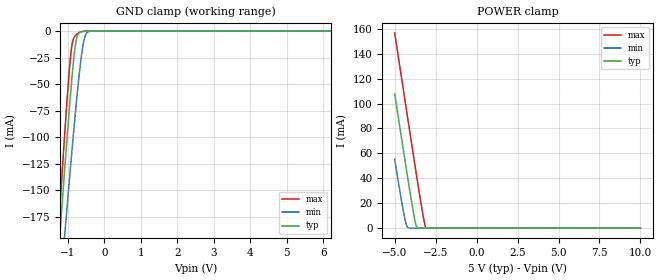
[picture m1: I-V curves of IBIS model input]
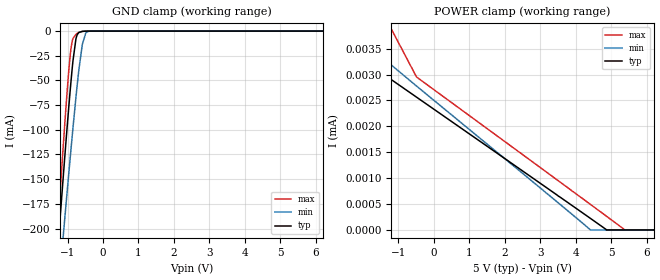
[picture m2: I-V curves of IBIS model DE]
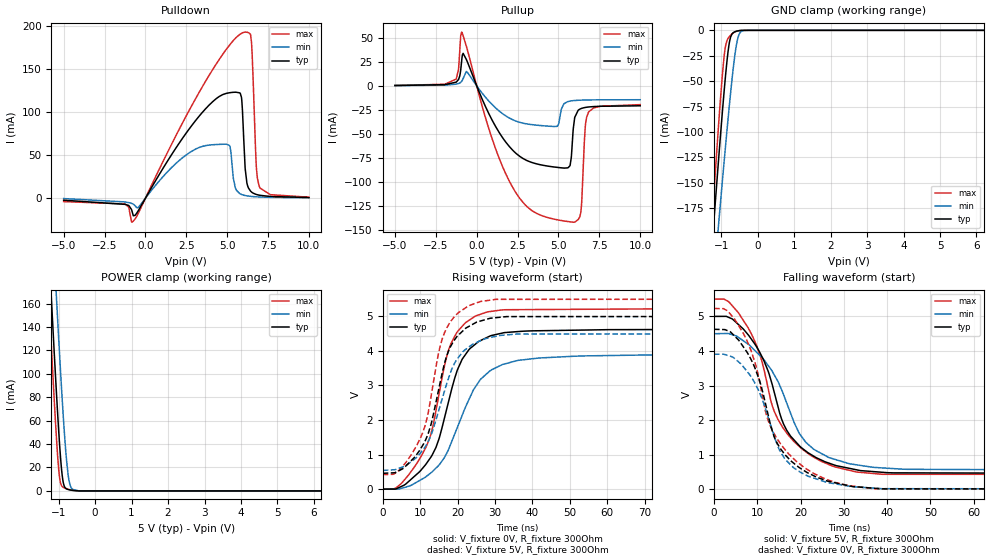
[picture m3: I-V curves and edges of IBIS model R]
|Texas Instruments Incorporated
| THVD1500 5-V RS-485 Transceivers With +/-16-kV IEC ESD Protection
| Marketing part#   Digital Voltage Range   Package-type   #pins
| THVD1500D   4.5V-5.5V   SOIC   8
| THVD1500DGK   4.5V-5.5V   VSSOP   8
[IBIS Ver]   4.1
[File name]   thvd1500.ibs
[Date]   06/22/2017
[File Rev]   1.0
[Source]
| Texas Instruments Incorporated.
| Analog-eLab Design Center, HPA
| 12500 TI Blvd
| Dallas, TX -75243
[Notes]
| Rev 1.0: 06/22/2017
| - Initial version of the model
| - Model generated from simulations in SPECTRE
| - Model matched to SPICE simulation
| - C_comp although listed in numerical order of value are
|   obtained from varying PVT conditions. For PVT conditions for
|   each specific value refer the buffer description under
|   respective [Model]. IBIS model user is responsible for using
|   appropriate C_comp to simulate for Signal Integrity.
| - Warnings regarding combined Non-monotonicity of various models
|   have been reviewed and considered minor and can be ignored.
| - Connect 1uF capacitor at the common mode node or bias the common mode
|   node to common mode voltage (Vcm= Vdd/2) for "diff" model.
[Disclaimer]
| This model is designed as an aid for customers of Texas Instruments.
| TI and its licensors and suppliers make no warranties, either expressed
| or implied, with respect to this  model, including the warranties of
| merchantability or fitness for a particular purpose. The model is
| provided solely on an "as is" basis. The entire risk as to its quality
| and performance is with the customer.
[Copyright]
(C) Copyright 2017 Texas Instruments Incorporated.All rights reserved.
|   THVD1500D
[Component]   THVD1500D
[Manufacturer]  TI
[Package]   |8 SOIC - D package
|   typ   min   max
R_pkg   0.10253625   0.06439   0.14266
L_pkg   2.75548625nH   2.22171nH   3.36255nH
C_pkg   0.4486575pF   0.38224pF   0.53208pF
[Pin]  signal_name model_name   R_pin   L_pin   C_pin
1   R   R   0.14266   3.36255nH   0.45815pF
2   _RE   input   0.12915   2.66262nH   0.38676pF
3   DE   DE   0.12314   2.56565nH   0.38224pF
4   D   input   0.13372   3.21721nH   0.45009pF
5   GND   gnd   0.0779   2.80108nH   0.51775pF
6   A   diff   0.06439   2.22171nH   0.42942pF
7   B   diff   0.06577   2.26041nH   0.43277pF
8   VCC   power   0.08356   2.95266nH   0.53208pF
[Diff Pin]  inv_pin  vdiff  tdelay_typ tdelay_min tdelay_max
6   7   0.2   NA   NA   NA
|   THVD1500DGK
[Component]   THVD1500DGK
[Manufacturer]  TI
[Package]   |8 VSSOP - DGK package
|   typ   min   max
R_pkg   0   0   0
L_pkg   0   0   0
C_pkg   0   0   0
[Pin]  signal_name model_name   R_pin   L_pin   C_pin
1   R   R   NA   NA   NA
2   _RE   input   NA   NA   NA
3   DE   DE   NA   NA   NA
4   D   input   NA   NA   NA
5   GND   gnd   NA   NA   NA
6   A   diff   NA   NA   NA
7   B   diff   NA   NA   NA
8   VCC   power   NA   NA   NA
[Diff Pin]  inv_pin  vdiff  tdelay_typ tdelay_min tdelay_max
6   7   0.2   NA   NA   NA
| Models and submodels in the file (4): input (Input), DE (Input), R (3-state), diff (I/O)
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|   input Model
[Model]   input
Model_type   Input
Vinl = 0.5
Vinh = 4.5
|   typ   min   max
C_comp   2.23689E-12   2.18605E-12   2.33152E-12
[Model spec]
|subparameter
Vinl   0.5   0.45   0.55
Vinh   4.5   4.05   4.95
| Where Nom  PVT is Nominal Process, 5V, 27C
|   Fast PVT is Strong Process,  5.5V, -40C
|   Slow PVT is Weak Process,   4.5, 150C
[Voltage Range]   5   4.5   5.5
|Junction Temperature
[Temperature Range]   27   150   -40
[Power Clamp Reference]   5   4.5   5.5
[GND Clamp Reference]   0   0   0
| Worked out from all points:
|   GND clamp passes 1 mA (typ) near -0.65 V on its own axis
|   POWER clamp passes 1 mA (typ) near -3.66 V on its own axis
[GND Clamp]
|   Voltage   I(typ)   I(min)   I(max)
-5V       -2.085A    -1.893A    -2.324A
-1.25V    -208.4mA   -261mA     -185mA
-1.13V    -151.6mA   -211.2mA   -120.8mA
-1.07V    -123.8mA   -186.6mA   -89.87mA
-965mV    -76.9mA    -144.2mA   -40.07mA
-905mV    -51.84mA   -120.5mA   -18.16mA
-845mV    -29.36mA   -97.32mA   -7.284mA
-770mV    -9.1mA     -69.52mA   -3.504mA
-635mV    -678.5uA   -25.82mA   -708.8uA
-530mV    -118.1uA   -5.338mA   -104.9uA
-410mV    -14.01uA   -325uA     -9.602uA
10V       0A         0A         0A
[POWER Clamp]
|   Voltage   I(typ)   I(min)   I(max)
-5V       107.7mA    55.36mA    156.7mA
-4.55V    69.33mA    19.37mA    117.8mA
-4.415V   57.93mA    9.756mA    106.2mA
-4.295V   47.87mA    3.03mA     95.86mA
-4.16V    36.66mA    210uA      84.27mA
-3.875V   13.93mA    182.7nA    59.93mA
-3.725V   3.778mA    29.3nA     47.22mA
-3.605V   201.6uA    20.98nA    37.14mA
-3.275V   0A         7.077nA    10.49mA
-3.17V    0A         3.417nA    3.331mA
-3.08V    0A         522.7pA    241.1uA
10V       0A         0A         0A
|   DE Model
[Model]   DE
Model_type   Input
Vinl = 0.5
Vinh = 4.5
|   typ   min   max
C_comp   2.23689E-12   2.18605E-12   2.33152E-12
[Model spec]
|subparameter
Vinl   0.5   0.45   0.55
Vinh   4.5   4.05   4.95
| Where Nom  PVT is Nominal Process, 5V, 27C
|   Fast PVT is Strong Process,  5.5V, -40C
|   Slow PVT is Weak Process,   4.5, 150C
[Voltage Range]   5   4.5   5.5
|Junction Temperature
[Temperature Range]   27   150   -40
[Power Clamp Reference]   5   4.5   5.5
[GND Clamp Reference]   0   0   0
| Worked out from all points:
|   GND clamp passes 1 mA (typ) near -0.64 V on its own axis
[GND Clamp]
|   Voltage   I(typ)   I(min)   I(max)
-3.5V     -1.328A    -1.234A    -1.462A
-1.28V    -222.7mA   -273.5mA   -201.3mA
-1.088V   -132.1mA   -193.9mA   -99.04mA
-992mV    -88.68mA   -155mA     -52.01mA
-920mV    -57.92mA   -126.3mA   -22.8mA
-860mV    -34.63mA   -103mA     -8.912mA
-764mV    -8.061mA   -67.37mA   -3.317mA
-680mV    -1.448mA   -39.02mA   -1.343mA
-584mV    -294.7uA   -13.67mA   -295.3uA
-488mV    -54.4uA    -2.137mA   -42.87uA
-380mV    -6.239uA   -154.1uA   -3.22uA
8.5V      0A         0A         0A
[POWER Clamp]
|   Voltage   I(typ)   I(min)   I(max)
-3.5V     7.22uA     4.553uA    28.19mA
-3.164V   3.836uA    4.309uA    2.93mA
-2.984V   3.751uA    4.202uA    6.205uA
-488mV    2.563uA    2.778uA    2.952uA
4.408V    226.7nA    4.981nA    497.3nA
4.876V    139pA      0A         261nA
5.404V    0A         0A         0A
8.5V      0A         0A         0A
|   R Model
[Model]   R
Model_type   3-state
Polarity   Non-Inverting
Vmeas = 2.5
Vref = 0
Cref = 2pF
Rref = 100000
|   typ   min   max
C_comp   3.78133E-12   3.67829E-12   3.86963E-12
| Where Nom  PVT is Nominal Process, 5V, 27C
|   Fast PVT is Strong Process,  5.5V, -40C
|   Slow PVT is Weak Process,   4.5, 150C
[Voltage Range]   5   4.5   5.5
|Junction Temperature
[Temperature Range]   27   150   -40
[Pullup Reference]   5   4.5   5.5
[Pulldown Reference]   0   0   -0
[Power Clamp Reference]   5   4.5   5.5
[GND Clamp Reference]   0   0   0
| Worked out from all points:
|   slope of the pulldown table from 0 to 0.75 V, typ, clamps not added: 30.6 ohm
|   slope of the pullup table from 0 to 0.75 V, typ, clamps not added: 25.6 ohm
|   GND clamp passes 1 mA (typ) near -0.60 V on its own axis
|   POWER clamp passes 1 mA (typ) near -0.71 V on its own axis
|   falling waveform, V_fixture 5V, R_fixture 300Ohm: 20-80 % time 8.94ns typ, 9.65ns min, 9.39ns max; typ from 5 V to 0.459 V
|   rising waveform, V_fixture 0V, R_fixture 300Ohm: 20-80 % time 8.13ns typ, 10.2ns min, 7.4ns max; typ from 0 V to 4.63 V
|   rising waveform, V_fixture 5V, R_fixture 300Ohm: 20-80 % time 6.78ns typ, 7.64ns min, 6.49ns max; typ from 0.459 V to 5 V
|   falling waveform, V_fixture 0V, R_fixture 300Ohm: 20-80 % time 8.18ns typ, 7.91ns min, 9.06ns max; typ from 4.63 V to 0 V
[Pulldown]
|   Voltage   I(typ)   I(min)   I(max)
-5V       -2.285mA   -396.6uA   -3.911mA
-740mV    -20.39mA   -6.868mA   -26.54mA
4.735V    120.5mA    62.74mA    167.5mA
5.17V     122.7mA    60.06mA    178.6mA
5.5V      123.2mA    12.2mA     185.8mA
5.8V      122mA      5.077mA    190.7mA
5.905V    111.2mA    4.177mA    191.9mA
6.1V      34.79mA    3.13mA     193.1mA
6.49V     7.213mA    2.073mA    180.9mA
6.775V    4.462mA    1.659mA    39.69mA
6.955V    3.589mA    1.472mA    14.28mA
10V       821.4uA    503.4uA    1.196mA
[GND Clamp]
|   Voltage   I(typ)   I(min)   I(max)
-5V       -2.098A    -1.919A    -2.329A
-1.445V   -305.1mA   -348.1mA   -293.5mA
-1.25V    -210.4mA   -265mA     -186.2mA
-1.235V   -203.2mA   -258.6mA   -178mA
-1.07V    -125.5mA   -189.5mA   -91.17mA
-965mV    -78.34mA   -146.6mA   -41.78mA
-905mV    -53.2mA    -122.6mA   -20.57mA
-770mV    -10.57mA   -70.95mA   -5.896mA
-605mV    -1.093mA   -18.95mA   -1.249mA
-500mV    -276.7uA   -3.145mA   -267.2uA
-365mV    -21.88uA   -163.3uA   -12.63uA
10V       0A         0A         0A
[Pullup]
|   Voltage   I(typ)   I(min)   I(max)
-5V       291.5uA    198.8uA    370.4uA
-1.25V    3.835mA    1.712mA    7.075mA
-920mV    25.99mA    4.642mA    55.98mA
2.215V    -67.34mA   -35.47mA   -106.3mA
4.915V    -84.98mA   -42.24mA   -139.6mA
5.575V    -85.45mA   -16.44mA   -141.4mA
5.785V    -74.76mA   -15.7mA    -141.9mA
5.905V    -44.88mA   -15.45mA   -142.1mA
6.37V     -23.82mA   -14.95mA   -132mA
6.64V     -22.56mA   -14.81mA   -42.7mA
6.835V    -22.09mA   -14.74mA   -27.57mA
10V       -20.84mA   -14.52mA   -19.61mA
[POWER Clamp]
|   Voltage   I(typ)   I(min)   I(max)
-5V       2.649A     2.722A     2.615A
-1.415V   296.9mA    380.3mA    256.3mA
-1.25V    194.4mA    278mA      153.3mA
-1.175V   149mA      232.4mA    108.2mA
-1.07V    88.28mA    170mA      49.46mA
-995mV    48.91mA    127.1mA    16.77mA
-890mV    10.01mA    71.37mA    3.387mA
-815mV    2.435mA    37.41mA    2.238mA
-740mV    1.209mA    13.41mA    1.44mA
-635mV    534.1uA    1.704mA    595.4uA
-455mV    35.24uA    93.8uA     20.17uA
10V       0A         0A         0A
[Ramp]
R_load = 300
|   typ   min   max
dV/dt_r   2.77599/8.07686e-09   2.34441/1.00809e-08   3.13711/7.35871e-09
dV/dt_f   2.72458/8.82592e-09   2.37427/9.60233e-09   3.04734/9.36697e-09
[Falling Waveform]
V_fixture = 5V
V_fixture_min = 4.5V
V_fixture_max = 5.5V
R_fixture = 300Ohm
C_fixture = 0F
|   Time   V(typ)   V(min)   V(max)
0s        5V         4.5V       5.5V
3.459ns   4.969V     4.5V       5.418V
9.378ns   4.212V     4.023V     4.29V
11.1ns    3.831V     3.808V     3.686V
13.47ns   3.024V     3.41V      2.414V
17.05ns   1.658V     2.413V     1.583V
19.75ns   1.253V     1.606V     1.232V
23.09ns   950.6mV    1.149V     922.5mV
32.93ns   560.1mV    704.2mV    496.1mV
300ns     459mV      542.9mV    421.1mV
[Rising Waveform]
V_fixture = 0V
V_fixture_min = 0V
V_fixture_max = 0V
R_fixture = 300Ohm
C_fixture = 0F
|   Time   V(typ)   V(min)   V(max)
0s        2.117nV    112.4nV    1.611nV
4.8ns     69.63mV    18.41mV    147.5mV
10.17ns   542.3mV    270mV      930.7mV
12.68ns   895.8mV    454.9mV    1.518V
14.81ns   1.385V     670.3mV    2.608V
17.23ns   2.377V     1.067V     3.891V
19.73ns   3.376V     1.728V     4.52V
28.01ns   4.396V     3.361V     5.13V
54.25ns   4.604V     3.856V     5.205V
300ns     4.627V     3.907V     5.229V
[Rising Waveform]
V_fixture = 5V
V_fixture_min = 4.5V
V_fixture_max = 5.5V
R_fixture = 300Ohm
C_fixture = 0F
|   Time   V(typ)   V(min)   V(max)
0s        459mV      542.9mV    421.1mV
4.505ns   543.8mV    609.1mV    558.9mV
9.811ns   1.112V     1.007V     1.422V
11.35ns   1.399V     1.226V     1.841V
12.89ns   1.865V     1.566V     2.667V
14.87ns   2.841V     2.24V      3.909V
16.52ns   3.636V     2.839V     4.527V
19.75ns   4.404V     3.746V     5.056V
26.2ns    4.867V     4.298V     5.431V
300ns     5V         4.5V       5.5V
[Falling Waveform]
|Gnd
V_fixture = 0V
V_fixture_min = 0V
V_fixture_max = 0V
R_fixture = 300Ohm
C_fixture = 0F
|   Time   V(typ)   V(min)   V(max)
0s        4.627V     3.907V     5.229V
3.211ns   4.583V     3.869V     5.152V
8.033ns   3.879V     3.349V     4.175V
10.45ns   3.174V     2.813V     3.17V
12.58ns   2.109V     2.061V     1.965V
13.9ns    1.518V     1.544V     1.609V
15.6ns    1.131V     1.034V     1.271V
21.74ns   467.6mV    375.8mV    557.6mV
31.15ns   98.82mV    86.88mV    99.02mV
300ns     3.499nV    113.7nV    2.551nV
